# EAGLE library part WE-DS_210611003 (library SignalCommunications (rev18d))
WE-DS D-SUB-Filter, Solder Pin Straight Characteristics Standard type filtered with 1000 pF High attenuation: max. ≥ 40 dB @ 180 MHz Choice of UNC 4/40 or through hole Rated voltage: 100 VDC Rated current @ 20 ºC: 5 A Withstand voltage: 250 VRMS Insulation resistance: min. 1000 MΩ Operating temperature: –55 ºC to +125 ºC Applications Filtering of interfaces External connection to -printer -sensor -display Details see: http://katalog.we-online.de/en/pbs/Filter_gerade Created on 2015-05-04 2015 (C) Wurth Elektronik
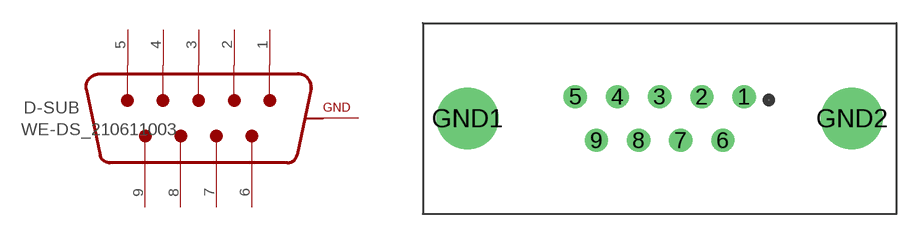
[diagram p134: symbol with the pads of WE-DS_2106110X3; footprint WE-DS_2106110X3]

Designator prefix D-SUB

## WE-DS_210611003 (WE-NUMBER: 210611003/9pins_female)  [WE-DS_2106110X3]
1  5  pas
2  4  pas
3  3  pas
4  2  pas
5  1  pas
6  9  pas
7  8  pas
8  7  pas
9  6  pas
GND1  GND  pwr
GND2  GND  pwr

## Footprint WE-DS_2106110X3 (pad centres in mm)
drill 1: 1 5.49,1.42; 2 2.74,1.42; 3 0,1.42; 4 -2.74,1.42; 5 -5.49,1.42; 6 4.11,-1.42; 7 1.37,-1.42; 8 -1.37,-1.42; 9 -4.11,-1.42
drill 3: GND1 -12.5,0; GND2 12.5,0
